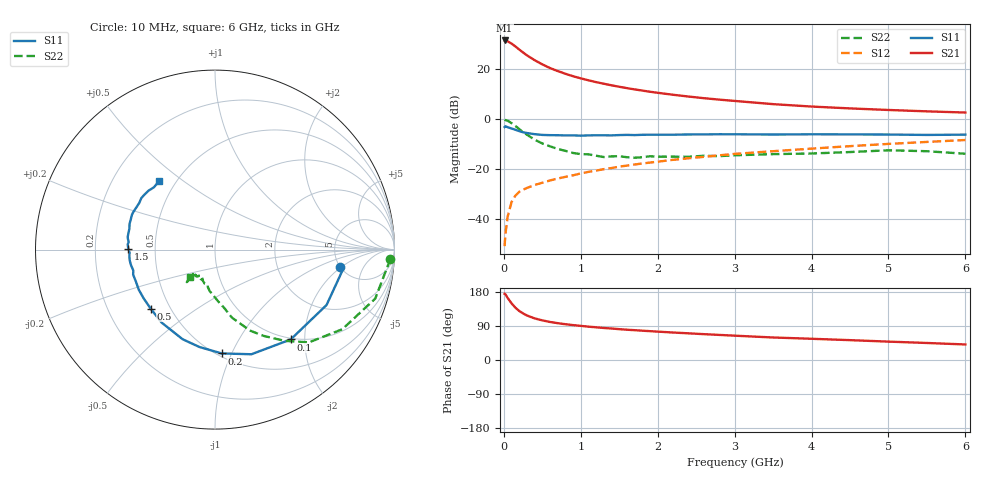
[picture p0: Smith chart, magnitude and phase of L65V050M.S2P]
!  INFINEON TECHNOLOGIES Small Signal Semiconductors
! BFR380L3 , Si-NPN RF-Transistor in TSLP-3-1
!  Vce=5 V,  Ic=50 mA
! Common Emitter S-Parameters:  07. March 2005
#  GHz  S  MA  R  50
! f  S11  S21  S12  S22
! GHz  Mag  Ang  Mag  Ang  Mag  Ang  Mag  Ang
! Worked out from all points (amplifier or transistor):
!   36 points, 10 MHz to 6 GHz, reference 50 ohm
!   highest |S21| = 31.5 dB at 10 MHz (marker M1)
!   |S21| within 3 dB of that: start of sweep to 174.4 MHz
!   unconditionally stable (mu >= 1): 1.686 GHz to 1.791 GHz; 1.802 GHz to 4.799 GHz
!   at 250 MHz: K = 0.43, MSG = 27.4 dB, |S12| = -28.2 dB
!   at 1.4 GHz: K = 0.97, MSG = 16.5 dB, |S12| = -19.5 dB
!   at 6 GHz: K = 0.97, MSG = 5.5 dB, |S12| = -8.3 dB
!   S11 on the Smith chart (normalised r, x): 10 MHz: 4.97, -1.86; 100 MHz: 0.98, -1.71; 200 MHz: 0.53, -0.92; 500 MHz: 0.39, -0.34; 1.5 GHz: 0.35, +0.01; 6 GHz: 0.41, +0.41
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0.01  0.7009 -7.8  37.68 174.7  0.0029 78.5  0.9783 -3.1
0.02  0.724 -8.1  37.26 173.5  0.005 88.6  0.9605 -6.8
0.05  0.694 -26.4  36.16 163.6  0.0114 78.9  0.9336 -17.0
0.1  0.6547 -49.9  32.62 149.6  0.0221 69.1  0.8368 -32.0
0.15  0.6174 -70.8  28.6 138.1  0.0297 62.0  0.736 -44.6
0.2  0.5797 -86.3  24.79 129.3  0.0354 58.9  0.6389 -52.7
0.25  0.5493 -99.2  21.67 122.9  0.039 55.7  0.5509 -60.7
0.3  0.5309 -109.9  19.01 117.5  0.0423 54.6  0.4926 -66.5
0.4  0.5037 -126.3  15.19 109.8  0.0485 54.5  0.3909 -76.0
0.5  0.4865 -137.4  12.53 104.6  0.0538 55.1  0.3285 -81.1
0.6  0.4814 -145.8  10.59 100.4  0.0598 56.5  0.2879 -86.7
0.8  0.4753 -158.0  8.128 94.4  0.0705 59.2  0.2335 -97.2
0.9  0.4769 -163.0  7.25 92.1  0.0757 60.8  0.2119 -100.9
1.1  0.476 -169.6  6.008 88.0  0.0887 62.5  0.199 -106.5
1.5  0.4833 179.3  4.468 81.4  0.1127 64.4  0.1826 -116.3
1.8  0.4891 172.9  3.749 77.3  0.1306 65.0  0.1739 -121.7
2.2  0.491 166.3  3.093 72.5  0.1545 65.5  0.1788 -125.0
2.8  0.5018 157.2  2.471 66.2  0.19 65.6  0.1831 -132.2
3.5  0.4957 148.5  2.007 59.4  0.2299 63.7  0.201 -131.4
4.5  0.4987 142.3  1.649 52.4  0.2902 62.2  0.2212 -131.2
5.5  0.4861 134.4  1.44 44.9  0.3524 58.7  0.2297 -130.8
6  0.4926 129.3  1.363 41.0  0.385 56.7  0.2043 -132.0
